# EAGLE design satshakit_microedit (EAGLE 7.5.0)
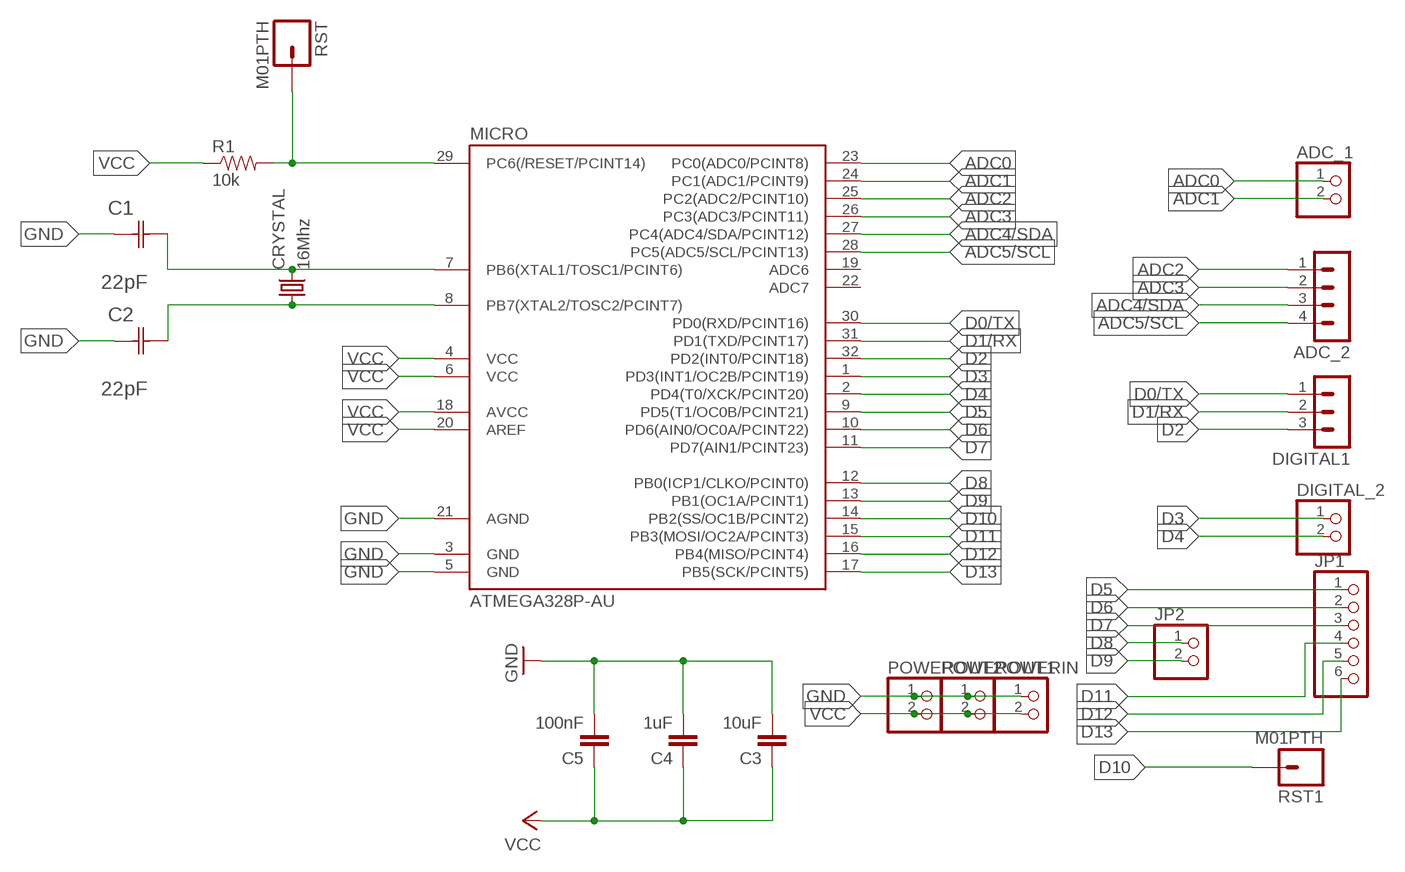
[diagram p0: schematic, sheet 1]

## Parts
ADC_1  PINHD-1X2  [1X02]
ADC_2  MA04-1  [MA04-1]
C1  22pF  0612ZC225MAT2A  [CAPC3216X178N]
C2  22pF  0612ZC225MAT2A  [CAPC3216X178N]
C3  10uF  CAP1206  [1206]
C4  1uF  CAP1206  [1206]
C5  100nF  CAP1206  [1206]
CRYSTAL  16Mhz  CSM-7X-DU  [CSM-7X-DU]
DIGITAL1  MA03-1  [MA03-1]
DIGITAL_2  PINHD-1X2  [1X02]
JP1  PINHD-1X6  [1X06]
JP2  PINHD-1X2  [1X02]
MICRO  ATMEGA328P-AU  ATMEGA48/88/168-AU  [TQFP32-08]
POWERIN  PINHD-1X2  [1X02]
POWEROUT1  PINHD-1X2  [1X02]
POWEROUT2  PINHD-1X2  [1X02]
R1  10k  RESISTOR1206  [1206]
RST  M01PTH  [1X01]
RST1  M01PTH  [1X01]

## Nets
ADC0: ADC_1.1 MICRO.23(PC0(ADC0/PCINT8))
ADC1: ADC_1.2 MICRO.24(PC1(ADC1/PCINT9))
ADC2: ADC_2.1 MICRO.25(PC2(ADC2/PCINT10))
ADC3: ADC_2.2 MICRO.26(PC3(ADC3/PCINT11))
ADC4/SDA: ADC_2.3 MICRO.27(PC4(ADC4/SDA/PCINT12))
ADC5/SCL: ADC_2.4 MICRO.28(PC5(ADC5/SCL/PCINT13))
D0/TX: DIGITAL1.1 MICRO.30(PD0(RXD/PCINT16))
D1/RX: DIGITAL1.2 MICRO.31(PD1(TXD/PCINT17))
D2: DIGITAL1.3 MICRO.32(PD2(INT0/PCINT18))
D3: DIGITAL_2.1 MICRO.1(PD3(INT1/OC2B/PCINT19))
D4: DIGITAL_2.2 MICRO.2(PD4(T0/XCK/PCINT20))
D5: JP1.1 MICRO.9(PD5(T1/OC0B/PCINT21))
D6: JP1.2 MICRO.10(PD6(AIN0/OC0A/PCINT22))
D7: JP1.3 MICRO.11(PD7(AIN1/PCINT23))
D8: JP2.1 MICRO.12(PB0(ICP1/CLKO/PCINT0))
D9: JP2.2 MICRO.13(PB1(OC1A/PCINT1))
D10: MICRO.14(PB2(SS/OC1B/PCINT2)) RST1.1
D11: JP1.4 MICRO.15(PB3(MOSI/OC2A/PCINT3))
D12: JP1.5 MICRO.16(PB4(MISO/PCINT4))
D13: JP1.6 MICRO.17(PB5(SCK/PCINT5))
GND: C1.1(C1) C2.1(C1) C3.2 C4.2 C5.2 MICRO.3(GND) MICRO.5(GND) MICRO.21(AGND) POWERIN.1 POWEROUT1.1 POWEROUT2.1
N$2: C1.2(C2) CRYSTAL.2 MICRO.7(PB6(XTAL1/TOSC1/PCINT6))
N$3: MICRO.29(PC6(/RESET/PCINT14)) R1.2 RST.1
N$9: C2.2(C2) CRYSTAL.1 MICRO.8(PB7(XTAL2/TOSC2/PCINT7))
VCC: C3.1 C4.1 C5.1 MICRO.4(VCC) MICRO.6(VCC) MICRO.18(AVCC) MICRO.20(AREF) POWERIN.2 POWEROUT1.2 POWEROUT2.2 R1.1
Unconnected: MICRO.19(ADC6) MICRO.22(ADC7)

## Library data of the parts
ADC_1 DIGITAL_2 JP2 POWERIN POWEROUT1 POWEROUT2 = pinhead:PINHD-1X2: PIN HEADER
ADC_2 = con-lstb:MA04-1: PIN HEADER; OC_FARNELL: unknown; OC_NEWARK: unknown
C1 C2 = AVX_By_element14_Batch_1:0612ZC225MAT2A: Capacitor 1206; MPN: 0612ZC225MAT2A; OC_FARNELL: -; OC_NEWARK: 12N3209; SUPPLIER: AVX; TOLERANCE: ±20%; VALUE: 2.2µF; VOLTAGERATING: 10V
C3-C5 = 01_SparkFun:CAP: Capacitor
CRYSTAL = 01_FAB_Hello:CSM-7X-DU: SMD CRYSTAL; OC_FARNELL: unknown; OC_NEWARK: unknown
DIGITAL1 = con-lstb:MA03-1: PIN HEADER; OC_FARNELL: unknown; OC_NEWARK: unknown
JP1 = pinhead:PINHD-1X6: PIN HEADER
MICRO = atmega8:ATMEGA48/88/168
R1 = 01_SparkFun:RESISTOR: Resistor
RST RST1 = 01_SparkFun:M01: Header 1

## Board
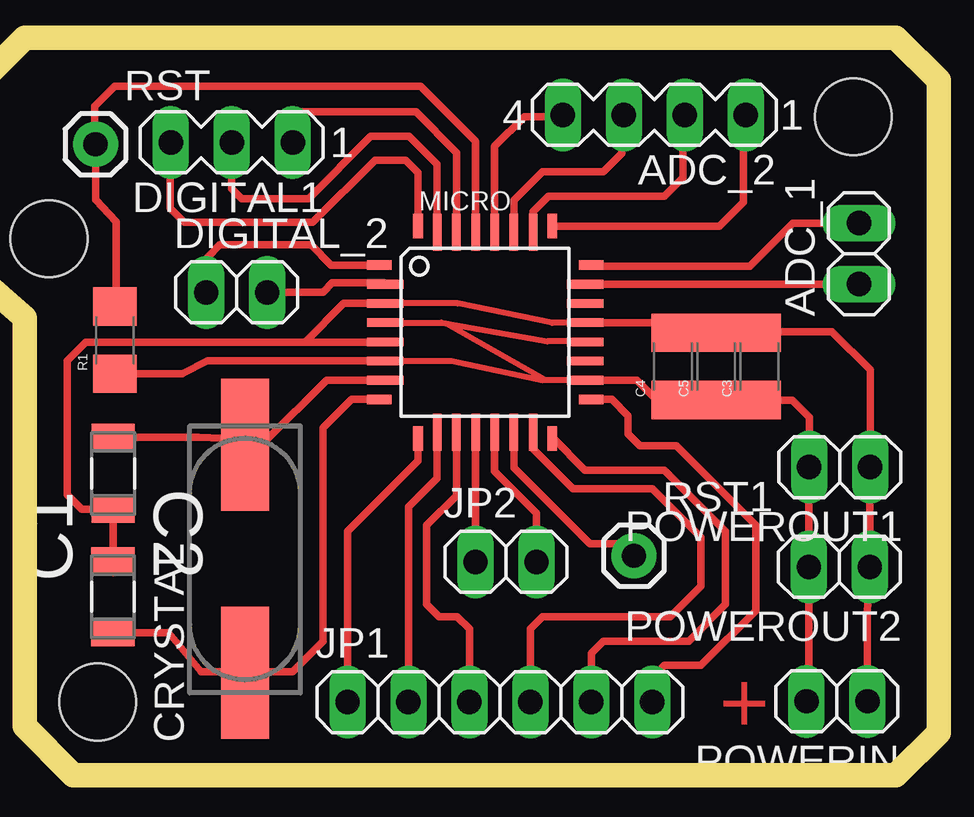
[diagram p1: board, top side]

No outline drawn. Coordinates in mm, seen from the top.
Copper layers (1*16): Top 0.035mm / dielectric 1.5mm / Bottom 0.035mm
Design rules "default": minimum track width 10mil, minimum drill 24mil, track to track 8mil, track to pad 8mil, pad to pad 8mil, via to via 8mil, smd to smd 8mil, copper to edge 40mil, drill to drill 8mil, minimum pad ring 10mil, minimum via ring 8mil, stop-mask expansion 4mil, vias tented up to drill 0mil, thermal gap 10mil
Holes 3.2 mm at 45.21,32.77 11.68,27.69 13.72,8.38
Milling: 10 lines

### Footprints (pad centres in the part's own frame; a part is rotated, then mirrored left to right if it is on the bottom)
1X02 = drill 1.016 long: 1 -1.27,0; 2 1.27,0
MA04-1 = drill 1.016 long: 1 -3.81,0; 2 -1.27,0; 3 1.27,0; 4 3.81,0
CAPC3216X178N = smd 1.118 x 1.803: 1 -1.499,0; 2 1.499,0
1206 = smd 1.6 x 1.8: 1 -1.4,0; 2 1.4,0
CSM-7X-DU = smd 5.5 x 2: 1 -4.75,0; 2 4.75,0
MA03-1 = drill 1.016 long: 1 -2.54,0; 2 0,0; 3 2.54,0
1X06 = drill 1.016 long: 1 -6.35,0; 2 -3.81,0; 3 -1.27,0; 4 1.27,0; 5 3.81,0; 6 6.35,0
TQFP32-08 = smd 1.016 x 0.406: 1 -4.42,2.8; 8 -4.42,-2.8; 17 4.42,-2.8; 24 4.42,2.8 | smd 1.524 x 0.356: 2 -4.166,2; 3 -4.166,1.2; 4 -4.166,0.4; 5 -4.166,-0.4; 6 -4.166,-1.2; 7 -4.166,-2; 18 4.166,-2; 19 4.166,-1.2; 20 4.166,-0.4; 21 4.166,0.4; 22 4.166,1.2; 23 4.166,2 | smd 0.406 x 1.016: 9 -2.8,-4.42; 16 2.8,-4.42; 25 2.8,4.42; 32 -2.8,4.42 | smd 0.356 x 1.524: 10 -2,-4.166; 11 -1.2,-4.166; 12 -0.4,-4.166; 13 0.4,-4.166; 14 1.2,-4.166; 15 2,-4.166; 26 2,4.166; 27 1.2,4.166; 28 0.4,4.166; 29 -0.4,4.166; 30 -1.2,4.166; 31 -2,4.166
1X01 = drill 1.016 pad 1.88: 1 0,0

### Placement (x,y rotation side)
ADC_1  45.45,27.07 90 top
ADC_2  36.92,32.85 180 top
C1  14.36,17.91 90 top
C2  14.35,12.77 270 top
C3  41.3,22.37 90 top
C4  37.69,22.37 90 top
C5  39.49,22.37 90 top
CRYSTAL  19.85,14.34 90 top
DIGITAL1  19.3,31.7 180 top
DIGITAL_2  19.51,25.45 0 top
JP1  30.48,8.38 0 top
JP2  30.73,14.22 0 top
MICRO  29.87,23.79 0 top
POWERIN  44.53,8.41 180 top
POWEROUT1  44.64,18.17 180 top
POWEROUT2  44.63,14.01 180 top
R1  14.43,23.46 90 top
RST  13.62,31.62 0 top
RST1  36.07,14.48 0 top

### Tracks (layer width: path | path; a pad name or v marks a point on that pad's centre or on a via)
ADC0
  Top 0.305: ADC_1.1 MICRO.23
ADC1
  Top 0.305: ADC_1.2 42.69,28.34 40.89,26.54 34.33,26.54 MICRO.24
ADC2
  Top 0.305: MICRO.25 39.64,28.21 40.64,29.21 40.64,32.76 ADC_2.1
ADC3
  Top 0.305: MICRO.26 31.86,28.82 32.51,29.46 37.34,29.46 38.1,30.23 38.1,32.76 ADC_2.2
ADC4/SDA
  Top 0.305: MICRO.27 31.07,29.29 32.26,30.48 34.8,30.48 35.56,31.24 35.56,32.76 ADC_2.3
ADC5/SCL
  Top 0.305: MICRO.28 30.27,31.54 31.5,32.77 33.02,32.77 ADC_2.4
D0/TX
  Top 0.305: MICRO.30 28.66,31.28 26.98,32.97 21.84,32.97 DIGITAL1.1
D1/RX
  Top 0.305: MICRO.31 27.86,30.78 26.7,31.95 25.09,31.95 22.5,29.36 19.71,29.36 19.3,29.77 DIGITAL1.2
D2
  Top 0.305: MICRO.32 27.07,30.44 26.54,30.96 25.27,30.96 22.68,28.37 17.32,28.37 16.74,28.96 16.74,31.67 DIGITAL1.3
D3
  Top 0.305: MICRO.1 23.45,26.59 22.61,27.43 18.8,27.43 18.29,26.92 18.29,25.5 DIGITAL_2.1
D4
  Top 0.305: DIGITAL_2.2 23.1,25.45 23.5,25.84 25.64,25.84 MICRO.2
D5
  Top 0.305: MICRO.9 27.07,18.43 24.13,15.49 JP1.1
D6
  Top 0.305: MICRO.10 27.86,17.7 26.67,16.51 JP1.2
D7
  Top 0.305: MICRO.11 28.66,16.98 27.43,15.75 27.43,12.45 27.94,11.94 28.7,11.94 29.21,11.43 JP1.3
D8
  Top 0.305: MICRO.12 JP2.1
D9
  Top 0.305: MICRO.13 30.27,18 32,16.26 JP2.2
D10
  Top 0.305: MICRO.14 31.07,18.15 34.23,14.99 35.56,14.99 RST1.1
D11
  Top 0.305: MICRO.15 31.86,18.93 33.53,17.27 36.83,17.27 38.86,15.24 38.86,13.21 37.59,11.94 32.26,11.94 31.75,11.43 JP1.4
D12
  Top 0.305: MICRO.16 32.66,19.41 34.04,18.03 37.34,18.03 39.88,15.49 39.88,12.45 38.35,10.92 34.8,10.92 34.29,10.41 JP1.5
D13
  Top 0.305: MICRO.17 35.14,20.99 35.81,20.32 35.81,19.56 36.32,19.05 37.85,19.05 41.15,15.75 41.15,12.19 38.86,9.91 37.34,9.91 36.83,9.4 JP1.6
GND
  Top 0.254: MICRO.21 34.02,24.18 32.65,24.18 28.72,24.99 MICRO.3
  Top 0.305: MICRO.21 37.27,24.19 C4.2 C5.2 C3.2 41.34,23.81 44.32,23.81 45.91,22.22 POWEROUT1.1 45.9,17.4 POWEROUT2.1 45.8,12.14 POWERIN.1 | C2.1 14.36,13.77 C1.1 13.05,16.41 12.45,17.02 12.45,22.61 13.21,23.37 22.35,23.37 | 22.35,23.37 25.68,23.37 MICRO.5 | MICRO.3 23.97,24.99 22.35,23.37
  Top 0.406: 41.3,23.65 C3.2
N$2
  Top 0.305: MICRO.7 23.25,21.79 20.7,19.24 19.9,19.05 CRYSTAL.2 19.55,18.03 18.92,19.37 17.93,19.41 C1.2
N$3
  Top 0.305: MICRO.29 29.46,31.75 27.18,34.04 14.41,34.04 13.59,33.21 13.59,31.97 RST.1 13.62,29.3 14.48,28.38 14.48,24.9 R1.2 14.64,24.88
N$9
  Top 0.305: MICRO.8 24.29,20.99 23.11,19.81 23.11,10.92 21.84,9.65 19.91,9.65 CRYSTAL.1 19.79,9.65 18.03,9.65 16.67,11.27 C2.2
VCC
  Top 0.254: MICRO.20 33.42,23.39 33.42,23.41 32.46,23.41 28.22,24.16 | MICRO.4 28.05,24.19 28.22,24.16 | 26.39,22.6 28.47,22.6 32.28,21.79 MICRO.18 | MICRO.18 32.41,21.79 28.22,24.16
  Top 0.305: MICRO.18 | MICRO.20 33.42,23.41 | 34.03,21.76 MICRO.18 | 26.39,22.6 MICRO.6 25.68,22.61 18.29,22.61 17.23,22.06 R1.1 | MICRO.18 36.19,21.8 37.03,20.95 38.28,20.95 38.3,20.93 37.73,20.93 C4.1 C5.1 C3.1 41.31,20.95 42.67,20.95 43.37,20.25 POWEROUT1.2 43.36,17.4 POWEROUT2.2 43.36,9.53 POWERIN.2
  Top 0.406: 41.3,21.11 C3.1

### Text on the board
Top: +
